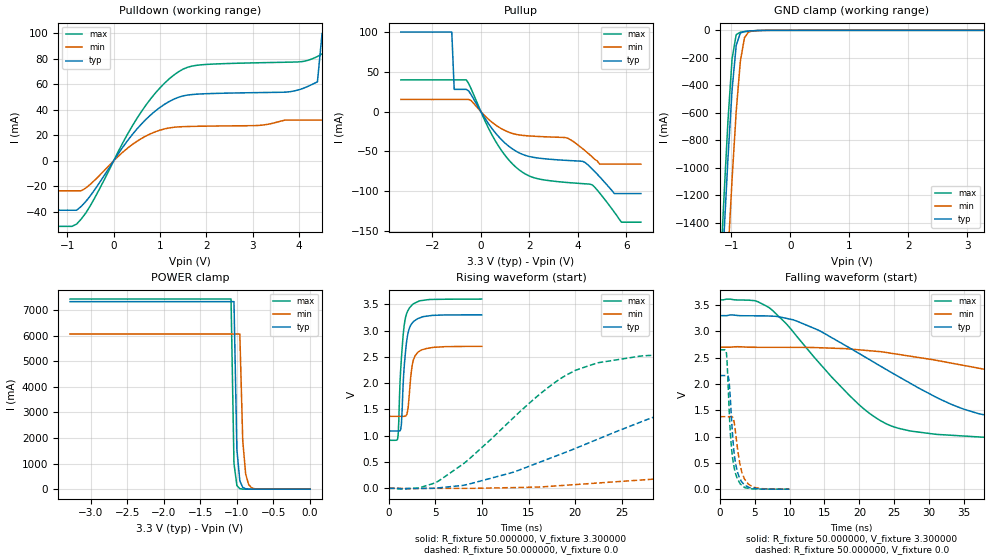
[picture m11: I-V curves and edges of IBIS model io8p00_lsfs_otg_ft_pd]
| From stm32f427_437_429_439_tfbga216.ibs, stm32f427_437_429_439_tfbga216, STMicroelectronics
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|   Model io8p00_lsfs_otg_ft_pd
[Model]  io8p00_lsfs_otg_ft_pd
Model_type I/O
Polarity   Non-Inverting
Enable   Active-Low
Vinl =   0.990000V
Vinh =   2.310000V
Vmeas =  1.650000V
Cref =   50.000000pF
Rref =   100.000000M
Vref =   0.0V
C_comp   8.196500pF   7.968500pF   8.492600pF
[Temperature Range]   25.000000   0.125000k   -40.000000
[Pullup Reference]   3.300000V   2.700000V   3.600000V
[Pulldown Reference]   0.0V   0.0V   0.0V
[POWER Clamp Reference]   3.300000V   2.700000V   3.600000V
[GND Clamp Reference]   0.0V   0.0V   0.0V
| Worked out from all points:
|   slope of the pulldown table from 0 to 0.495 V, typ, clamps not added: 20.1 ohm
|   slope of the pullup table from 0 to 0.495 V, typ, clamps not added: 21.8 ohm
|   GND clamp passes 1 mA (typ) near -0.52 V on its own axis
|   POWER clamp passes 1 mA (typ) near -0.81 V on its own axis
|   rising waveform, R_fixture 50.000000, V_fixture 3.300000: 20-80 % time 526ps typ, 500ps min, 529ps max; typ from 1.09 V to 3.3 V
|   rising waveform, R_fixture 50.000000, V_fixture 0.0: 20-80 % time 19.4ns typ, 47.3ns min, 10.3ns max; typ from 0 V to 2.16 V
|   falling waveform, R_fixture 50.000000, V_fixture 3.300000: 20-80 % time 18.4ns typ, 37.6ns min, 11.3ns max; typ from 3.3 V to 1.09 V
|   falling waveform, R_fixture 50.000000, V_fixture 0.0: 20-80 % time 845ps typ, 1.06ns min, 753ps max; typ from 2.16 V to 0 V
[Pulldown]
|Voltage   I(typ)   I(min)   I(max)
-3.3V     -38.65mA   -23.43mA   -51.3mA
-800mV    -38.65mA   -23.43mA   -49.55mA
600mV     28.88mA    17.56mA    38.65mA
1.4V      49.88mA    26.66mA    69.84mA
4.1V      56.96mA    32mA       77.99mA
4.4V      62mA       32mA       81.8mA
4.5V      100mA      32mA       83.9mA
4.7V      100mA      32mA       89mA
4.8V      100mA      32mA       100mA
5.1V      100mA      32mA       100mA
5.2V      1A         1A         100mA
6.6V      1A         1A         1A
[Pullup]
|Voltage   I(typ)   I(min)   I(max)
-3.3V     100mA      15.32mA    39.89mA
-1.2V     100mA      15.32mA    39.89mA
-1.1V     27.98mA    15.32mA    39.89mA
-600mV    27.98mA    15.32mA    39.89mA
500mV     -22.94mA   -14.36mA   -31.63mA
1.3V      -46.85mA   -27.39mA   -65.63mA
2.1V      -57.1mA    -30.77mA   -82.2mA
3.5V      -61.24mA   -32.71mA   -88.93mA
4.6V      -72.4mA    -57.1mA    -92.27mA
5.5V      -103mA     -66mA      -126.3mA
5.8V      -103mA     -66mA      -139mA
6.6V      -103mA     -66mA      -139mA
[GND_clamp]
|Voltage   I(typ)   I(min)   I(max)
-3.3V     -9.479A    -9.465A    -9.974A
-1.2V     -2.125A    -2.854A    -1.857A
-1.13V    -1.511A    -2.236A    -1.236A
-1.06V    -933.3mA   -1.641A    -660.9mA
-990mV    -433.3mA   -1.082A    -207mA
-920mV    -110.3mA   -591mA     -31.46mA
-850mV    -19.8mA    -226.8mA   -13.66mA
-780mV    -8.323mA   -53.94mA   -9.521mA
-710mV    -5.297mA   -11.95mA   -6.277mA
-640mV    -3.244mA   -4.292mA   -3.591mA
3.28V     81.28uA    57.87uA    93.98uA
[POWER_clamp]
|Voltage   I(typ)   I(min)   I(max)
-3.28V    7.328A     6.064A     7.43A
-1.08V    7.328A     6.064A     7.43A
-1.04V    7.328A     6.064A     1.015A
-1V       1.545A     6.064A     138.6mA
-960mV    325.6mA    6.064A     18.93mA
-920mV    68.64mA    1.89A      2.585mA
-880mV    14.47mA    589mA      353uA
-840mV    3.05mA     183.6mA    105.2uA
-800mV    642.9uA    57.21mA    105.2uA
-720mV    28.59uA    5.557mA    105.2uA
0V        0A         0A         0A
[Ramp]
| variable   typ   min   max
dV/dt_r  1.29569/19.42054n   0.82704/47.35804n   1.59013/10.26639n
dV/dt_f  1.32552/18.34344n   0.79752/37.70310n   1.61111/11.26081n
R_load = 50.000000
[Rising Waveform]
R_fixture= 50.000000
V_fixture= 3.300000
V_fixture_min= 2.700000
V_fixture_max= 3.600000
|time   V(typ)   V(min)   V(max)
0s        1.09V      1.369V     913.6mV
940.9ps   1.09V      1.369V     943.1mV
1.061ns   1.09V      1.369V     1.262V
1.281ns   1.132V     1.369V     2.293V
1.662ns   2.349V     1.37V      3.118V
1.942ns   2.836V     1.409V     3.337V
2.202ns   3.043V     1.802V     3.429V
2.503ns   3.142V     2.339V     3.487V
3.163ns   3.231V     2.595V     3.554V
9.97ns    3.299V     2.699V     3.599V
[Rising Waveform]
R_fixture= 50.000000
V_fixture= 0.0
V_fixture_min= 0.0
V_fixture_max= 0.0
|time   V(typ)   V(min)   V(max)
0s        8.71uV     4.057uV    76.57uV
5.506ns   12.07mV    -344.2uV   159.8mV
13.51ns   315.2mV    15.23mV    1.365V
20.02ns   759.2mV    71.83mV    2.243V
27.53ns   1.295V     164.1mV    2.522V
36.04ns   1.788V     306mV      2.603V
43.54ns   1.979V     443.5mV    2.626V
76.58ns   2.138V     1.046V     2.65V
104.1ns   2.157V     1.264V     2.65V
249.2ns   2.16V      1.378V     2.65V
[Falling Waveform]
R_fixture= 50.000000
V_fixture= 3.300000
V_fixture_min= 2.700000
V_fixture_max= 3.600000
|time   V(typ)   V(min)   V(max)
0s        3.299V     2.699V     3.599V
5.506ns   3.296V     2.697V     3.562V
11.01ns   3.197V     2.696V     2.91V
21.52ns   2.457V     2.631V     1.434V
31.03ns   1.744V     2.449V     1.042V
37.04ns   1.436V     2.301V     993.5mV
46.05ns   1.25V      2.087V     959.8mV
65.57ns   1.145V     1.677V     927.7mV
86.09ns   1.114V     1.51V      917mV
249.2ns   1.09V      1.369V     913.6mV
[Falling Waveform]
R_fixture= 50.000000
V_fixture= 0.0
V_fixture_min= 0.0
V_fixture_max= 0.0
|time   V(typ)   V(min)   V(max)
0s        2.16V      1.378V     2.65V
981ps     2.161V     1.378V     2.566V
1.321ns   2.074V     1.378V     1.615V
1.461ns   1.844V     1.379V     1.209V
1.682ns   1.365V     1.38V      794.3mV
2.002ns   765.2mV    1.315V     459.4mV
2.503ns   351.8mV    825.7mV    205.4mV
3.183ns   134.9mV    313mV      73.61mV
4.084ns   41.13mV    97.78mV    17.55mV
9.97ns    8.71uV     4.057uV    76.57uV
